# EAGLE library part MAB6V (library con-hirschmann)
Female CONNECTOR 6 pins with shield, vertical (DIN 45322)
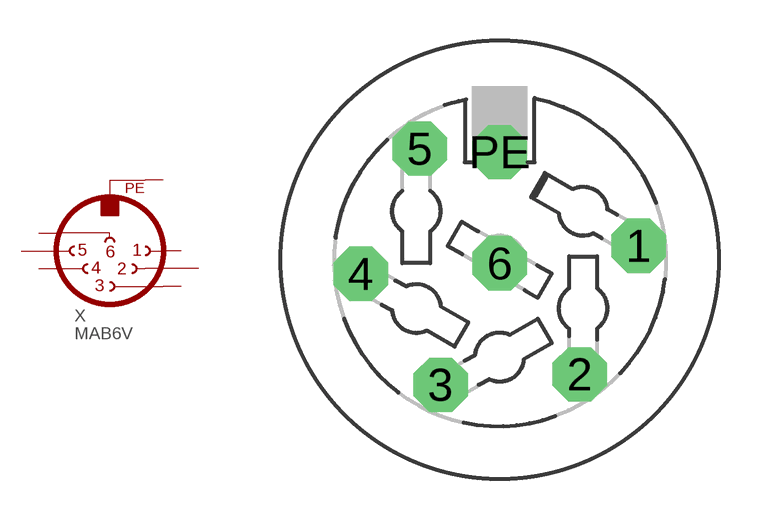
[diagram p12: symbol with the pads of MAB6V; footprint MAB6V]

Designator prefix X

## MAB6V (OC_FARNELL: unknown; OC_NEWARK: unknown)  [MAB6V]
1  1  pas
2  2  pas
3  3  pas
4  4  pas
5  5  pas
6  6  pas
PE  PE  pwr

## Footprint MAB6V (pad centres in mm)
Female CONNECTOR 6 pins with shield, vertical (DIN 45322)
drill 1.321 octagon: 1 5.08,0.508; 2 2.921,-4.191; 3 -2.159,-4.572; 4 -5.08,-0.508; 5 -2.921,4.064; 6 0,-0.127; PE 0,3.937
